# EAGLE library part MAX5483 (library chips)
SPI Programmable Rheostat
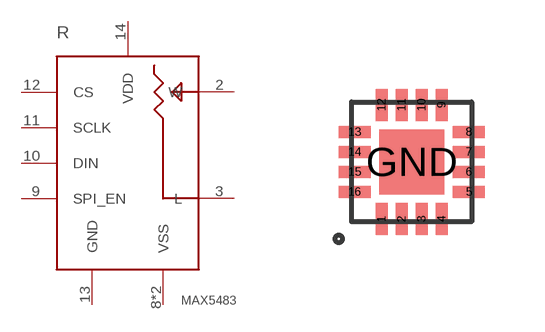
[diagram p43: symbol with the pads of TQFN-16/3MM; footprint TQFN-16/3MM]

Designator prefix R

## MAX5483 (DIGIKEY: MAX5483ETE+-ND)  [TQFN-16/3MM]
2  W
3  L
8  VSS
9  SPI_EN
10  DIN
11  SCLK
12  CS
13  GND
14  VDD
16  VSS

## Footprint TQFN-16/3MM (pad centres in mm)
smd 0.3 x 0.8: 1 -0.75,-1.43; 2 -0.25,-1.43; 3 0.25,-1.43; 4 0.75,-1.43; 9 0.75,1.43; 10 0.25,1.43; 11 -0.25,1.43; 12 -0.75,1.43
smd 0.8 x 0.3: 5 1.43,-0.75; 6 1.43,-0.25; 7 1.43,0.25; 8 1.43,0.75; 13 -1.43,0.75; 14 -1.43,0.25; 15 -1.43,-0.25; 16 -1.43,-0.75
smd 1.63 x 1.63: GND 0,0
